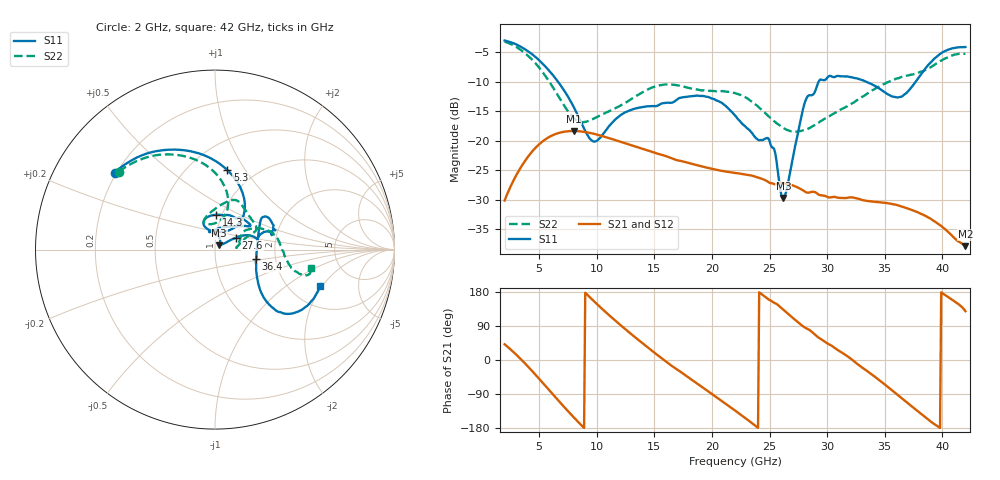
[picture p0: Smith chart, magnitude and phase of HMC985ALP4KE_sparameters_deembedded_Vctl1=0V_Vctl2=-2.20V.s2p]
!s2p File: Measurements: S11, S21, S12, S22
# GHz S dB R 50.0
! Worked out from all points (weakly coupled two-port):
!   401 points, 2 GHz to 42 GHz, reference 50 ohm
!   highest |S21| = -18.35 dB at 8 GHz (marker M1); lowest = -37.8 dB at 42 GHz (marker M2)
!   lowest |S11| = -29.7 dB at 26.2 GHz (marker M3), VSWR 1.07, Z = 52.3 + j2.43 ohm
!   |S11| at or under -10 dB: 6.629 GHz to 29.27 GHz (22.64 GHz wide, 126 % of centre); 33.37 GHz to 37.7 GHz (4.328 GHz wide, 12.2 % of centre)
!   |S22| runs from -18.5 to -3.2 dB; largest |S21 - S12| = 0.00041
!   S11 on the Smith chart (normalised r, x): 2 GHz: 0.19, +0.33; 5.3 GHz: 0.75, +0.83; 14.3 GHz: 0.94, +0.38; 27.6 GHz: 1.25, +0.17; 36.4 GHz: 1.58, -0.18; 42 GHz: 2.90, -1.91
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2  -3.04 142.5  -30.11 41.5  -30.11 41.5  -3.23 141.0
3.6  -4.33 113.5  -23.91 -3.6  -23.92 -3.7  -4.93 111.6
5.3  -6.96 81.2  -20.10 -60.0  -20.12 -60.0  -8.40 84.1
8  -14.29 47.5  -18.35 -151.2  -18.34 -151.2  -16.19 83.9
8.7  -17.14 52.3  -18.44 -173.2  -18.43 -173.2  -16.87 96.7
9.9  -20.10 88.6  -18.90 150.9  -18.89 150.9  -16.10 110.7
12.2  -15.50 112.3  -20.25 88.5  -20.28 88.4  -13.90 99.4
14.3  -14.21 88.3  -21.54 36.2  -21.53 36.2  -11.45 78.0
15.4  -13.94 73.2  -22.25 10.3  -22.22 10.3  -10.65 70.5
19.3  -12.45 34.2  -24.42 -74.7  -24.47 -74.8  -11.48 41.9
22  -15.72 52.3  -25.45 -133.2  -25.42 -133.2  -11.95 25.2
25  -20.03 98.6  -27.12 158.4  -27.14 158.4  -16.04 17.4
26.2  -29.66 45.0  -27.17 132.5  -27.22 132.4  -17.84 8.8
27.6  -17.38 29.7  -28.06 96.3  -28.08 96.3  -18.36 5.3
28.1  -13.31 20.9  -28.63 85.1  -28.65 85.2  -18.15 7.6
28.7  -12.27 13.0  -28.64 73.5  -28.62 73.5  -17.59 12.2
31  -9.06 23.3  -29.66 24.8  -29.63 24.7  -14.91 31.3
33.3  -9.94 34.2  -30.13 -25.4  -30.15 -25.5  -12.28 28.6
35.4  -12.27 12.1  -30.61 -74.3  -30.62 -74.2  -10.00 19.2
36.4  -12.58 -13.1  -31.08 -98.9  -31.06 -99.0  -9.24 13.2
39.5  -5.81 -43.4  -33.88 -172.9  -33.89 -173.2  -6.91 -14.0
42  -4.14 -19.0  -37.83 128.7  -37.80 128.8  -5.27 -10.8
